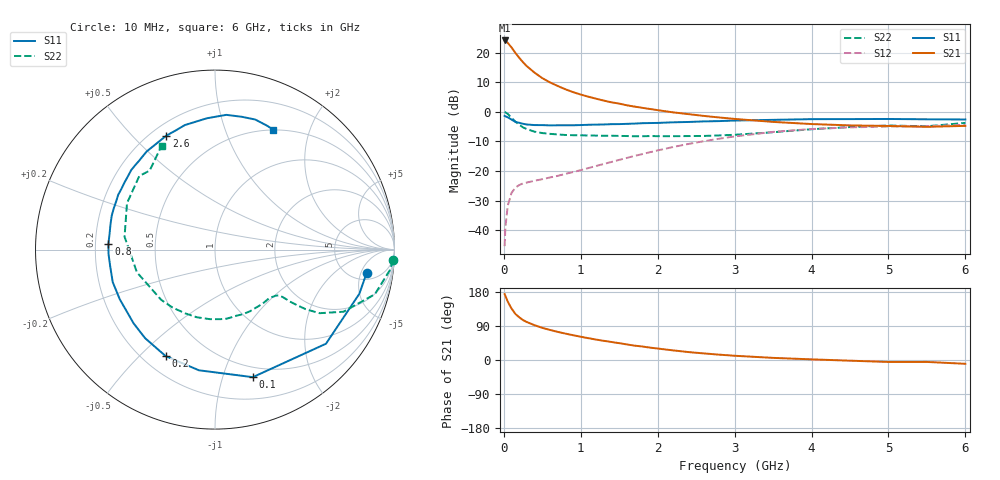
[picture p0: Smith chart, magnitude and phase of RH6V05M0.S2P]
! SIEMENS Small Signal Semiconductors
! BFR106
! Si NPN RF Bipolar Junction Transistor in SOT23
! VCE = 6 V  IC = 5 mA
! Common Emitter S-Parameters:  August  1996
# GHz  S  MA  R  50
!  f  S11  S21  S12  S22
! GHz  MAG  ANG  MAG  ANG  MAG  ANG  MAG  ANG
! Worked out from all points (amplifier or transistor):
!   36 points, 10 MHz to 6 GHz, reference 50 ohm
!   highest |S21| = 24.1 dB at 10 MHz (marker M1)
!   |S21| within 3 dB of that: start of sweep to 117.3 MHz
!   unconditionally stable (mu >= 1): 623 MHz to 1.867 GHz; 4.958 GHz to end of sweep
!   at 250 MHz: K = 0.50, MSG = 20.4 dB, |S12| = -24.2 dB
!   at 1.4 GHz: K = 1.13, MAG = 7.9 dB, |S12| = -16.9 dB
!   at 6 GHz: K = 1.02, MAG = -1.0 dB, |S12| = -4.4 dB
!   S11 on the Smith chart (normalised r, x): 10 MHz: 6.61, -6.35; 100 MHz: 0.40, -1.26; 200 MHz: 0.29, -0.60; 800 MHz: 0.25, +0.03; 2.6 GHz: 0.26, +0.63; 6 GHz: 0.50, +1.48
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0.01  0.8549 -8.7  16.06 173.8  0.0054 88.3  0.9936 -3.3
0.02  0.8411 -17.0  15.93 169.4  0.011 83.1  0.9809 -6.7
0.05  0.8108 -40.3  14.66 154.4  0.0257 69.9  0.9248 -15.6
0.1  0.7412 -73.5  12.23 135.8  0.0429 55.3  0.7954 -25.8
0.15  0.6784 -97.6  9.903 121.6  0.0525 46.8  0.682 -31.3
0.2  0.6539 -114.9  8.189 112.7  0.0582 42.8  0.6052 -33.3
0.25  0.6286 -128.3  6.861 105.2  0.062 39.9  0.5473 -34.2
0.3  0.6118 -137.9  5.89 100.0  0.0641 39.8  0.5106 -34.7
0.4  0.5984 -152.5  4.58 91.8  0.0687 40.4  0.4625 -35.0
0.5  0.5979 -162.4  3.71 84.9  0.073 42.4  0.4387 -35.6
0.6  0.5913 -171.1  3.146 79.3  0.0781 45.4  0.4255 -37.1
0.8  0.5947 176.9  2.408 69.7  0.0897 51.3  0.4071 -41.4
1.1  0.6056 161.9  1.801 57.5  0.1126 58.8  0.3994 -50.0
1.3  0.6128 153.9  1.548 50.6  0.1322 62.0  0.395 -56.6
1.6  0.6276 143.5  1.29 41.0  0.1671 64.5  0.3907 -67.9
2.2  0.6662 124.9  0.981 25.4  0.2549 62.3  0.3886 -94.3
2.6  0.6904 113.1  0.854 17.4  0.3195 57.0  0.3922 -115.1
3.5  0.7332 93.5  0.677 5.6  0.459 40.5  0.4531 -163.8
4.5  0.7549 78.5  0.591 -1.8  0.5468 20.3  0.5543 152.2
5  0.7586 72.8  0.578 -5.2  0.5661 11.8  0.5882 135.8
5.5  0.7489 67.4  0.559 -5.1  0.5727 7.5  0.5712 129.6
6  0.7434 64.0  0.58 -10.0  0.6039 -0.6  0.6513 117.1
